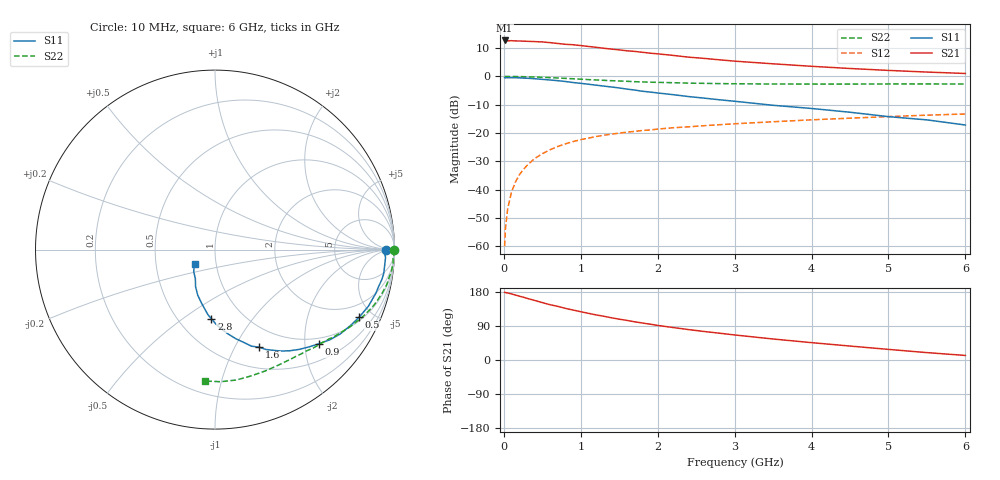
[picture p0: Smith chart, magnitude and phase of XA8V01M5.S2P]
! SIEMENS Discrete & RF Semiconductors
! BFY180
! Si NPN RF Bipolar Junction Transistor in MICRO-X
! VCE = 8 V  IC = 1.5 mA
! Common Emitter S-Parameters:  May  1997
# GHz  S  MA  R  50
!  f  S11  S21  S12  S22
! GHz  MAG  ANG  MAG  ANG  MAG  ANG  MAG  ANG
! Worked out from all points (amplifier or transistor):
!   36 points, 10 MHz to 6 GHz, reference 50 ohm
!   highest |S21| = 12.7 dB at 10 MHz (marker M1)
!   |S21| within 3 dB of that: start of sweep to 1.381 GHz
!   unconditionally stable (mu >= 1): 3.609 GHz to end of sweep
!   at 250 MHz: K = 0.09, MSG = 22.7 dB, |S12| = -33.0 dB
!   at 1.4 GHz: K = 0.56, MSG = 15.0 dB, |S12| = -20.4 dB
!   at 6 GHz: K = 1.06, MAG = 5.7 dB, |S12| = -13.3 dB
!   S11 on the Smith chart (normalised r, x): 10 MHz: 40, -4; 500 MHz: 1.18, -4.18; 900 MHz: 0.86, -2.31; 1.6 GHz: 0.74, -1.26; 2.8 GHz: 0.72, -0.65; 6 GHz: 0.79, -0.13
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0.01  0.9519 -0.3  4.321 178.6  0.001 89.2  0.995 -0.2
0.02  0.9437 -1.0  4.315 178.0  0.002 96.8  0.9985 -0.6
0.05  0.9513 -2.6  4.254 176.9  0.0046 86.3  0.9971 -1.5
0.1  0.9495 -5.1  4.283 174.3  0.0091 88.1  0.9931 -3.0
0.15  0.9496 -8.0  4.237 171.5  0.0135 85.6  0.9955 -4.4
0.3  0.929 -15.1  4.178 162.8  0.0266 79.5  0.9835 -8.7
0.5  0.8874 -25.1  4.07 151.5  0.043 73.4  0.9644 -14.2
0.6  0.8651 -29.3  3.957 145.9  0.0505 70.2  0.951 -16.8
0.8  0.8138 -38.1  3.697 136.3  0.0642 64.9  0.9234 -21.5
0.9  0.78 -42.3  3.629 131.8  0.0706 62.2  0.9082 -23.8
1.1  0.7278 -49.8  3.385 123.1  0.0812 57.8  0.8786 -27.8
1.4  0.6502 -59.7  3.039 111.4  0.0954 52.1  0.8401 -33.4
1.6  0.5966 -65.7  2.835 104.5  0.1034 49.2  0.8202 -36.6
1.7  0.5751 -69.3  2.768 100.8  0.1069 47.7  0.8072 -38.0
2  0.5102 -76.8  2.505 91.3  0.1174 44.1  0.7852 -42.4
2.2  0.476 -81.1  2.352 85.7  0.1238 41.7  0.7744 -45.2
2.6  0.4141 -89.4  2.084 75.3  0.1346 38.2  0.7542 -50.3
2.8  0.3867 -92.9  1.967 70.8  0.1401 36.7  0.7466 -52.8
3.5  0.3089 -103.9  1.67 55.4  0.158 31.2  0.7341 -61.3
4.5  0.2328 -117.7  1.381 36.8  0.1828 23.9  0.732 -74.0
5.5  0.1706 -134.1  1.194 19.5  0.2067 16.1  0.7367 -87.6
6  0.1384 -145.6  1.127 12.0  0.2168 12.0  0.7346 -94.5
